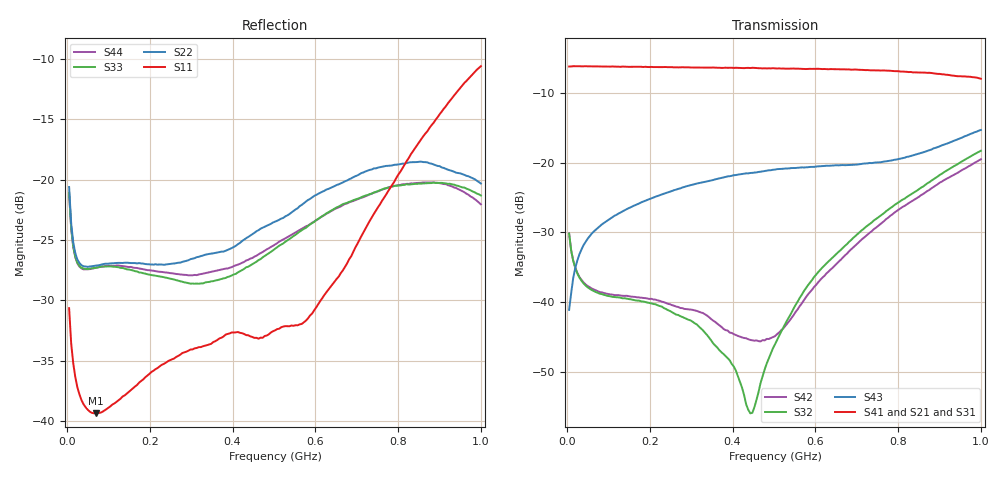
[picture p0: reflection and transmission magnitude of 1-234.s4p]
!Vector Network Analyzer,NA7684A,8000025053,DSP: 1.0.1
!Date: 2021-10-28 16:52
!Data & Calibration Information:
!Freq	S11:SOLT4(ON)	S12:SOLT4(ON)	S13:SOLT4(ON)	S14:SOLT4(ON)
!	S21:SOLT4(ON)	S22:SOLT4(ON)	S23:SOLT4(ON)	S24:SOLT4(ON)
!	S31:SOLT4(ON)	S32:SOLT4(ON)	S33:SOLT4(ON)	S34:SOLT4(ON)
!	S41:SOLT4(ON)	S42:SOLT4(ON)	S43:SOLT4(ON)	S44:SOLT4(ON)
# Hz S dB R 50
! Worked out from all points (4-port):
!   201 points, 5 MHz to 1 GHz, reference 50 ohm
!   strongest paths, dB at 5 MHz, 253.8 MHz, 502.5 MHz, 751.2 MHz, 1 GHz:
!     S41: -6.2, -6.3, -6.5, -6.8, -8.0
!     S21: -6.2, -6.3, -6.6, -6.9, -8.1
!     S31: -6.2, -6.4, -6.6, -7.0, -8.1
!     S43: -41.1, -24.1, -21.0, -20.0, -15.3
!     S32: -30.2, -41.4, -46.0, -27.9, -18.3
!     S42: -30.2, -40.4, -44.9, -29.1, -19.5
!   lowest |S11| = -39.4 dB at 69.67 MHz (marker M1), VSWR 1.02, Z = 50.3 + j1.05 ohm
!   |S11| at or under -10 dB: start of sweep to end of sweep
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5000000  -30.65 121.4  -6.17 0.4  -6.21 0.6  -6.23 0.4
         -6.19 0.2  -20.62 137.4  -30.14 -42.6  -30.16 -42.9
         -6.21 0.0  -30.16 -42.7  -21.08 137.8  -41.11 73.5
         -6.23 -0.2  -30.16 -42.8  -41.10 73.7  -21.14 137.7
6.9675e7  -39.35 75.3  -6.19 -15.5  -6.22 -15.6  -6.20 -15.4
          -6.19 -15.9  -27.12 176.5  -38.40 -20.9  -38.20 -26.0
          -6.21 -16.1  -38.54 -21.2  -27.30 174.8  -29.60 45.4
          -6.22 -16.1  -38.32 -26.0  -29.60 45.2  -27.30 176.2
3.18425e8  -33.88 -34.3  -6.38 -72.6  -6.40 -73.0  -6.36 -72.3
           -6.36 -73.0  -26.39 -164.5  -42.75 -29.5  -41.42 -63.8
           -6.39 -73.5  -43.48 -29.7  -28.62 -169.4  -22.94 27.5
           -6.37 -73.0  -41.36 -65.0  -22.94 27.1  -27.85 -168.5
4.47775e8  -33.03 -87.2  -6.49 -103.4  -6.50 -103.8  -6.46 -103.0
           -6.47 -103.8  -24.51 -155.5  -61.46 35.0  -45.19 -127.2
           -6.48 -104.5  -55.85 51.7  -27.00 -152.9  -21.41 17.5
           -6.42 -103.5  -45.45 -127.4  -21.47 17.2  -26.49 -155.4
4.97525e8  -32.56 -116.7  -6.52 -115.6  -6.55 -115.9  -6.48 -114.8
           -6.50 -116.0  -23.56 -154.0  -47.23 103.5  -44.85 -170.9
           -6.54 -116.7  -46.61 94.5  -25.86 -150.5  -20.97 14.3
           -6.47 -115.6  -45.02 -168.8  -21.02 13.7  -25.49 -152.7
5.9205e8  -31.10 -178.8  -6.66 -139.4  -6.67 -139.7  -6.56 -138.5
          -6.66 -140.1  -21.48 -158.5  -36.77 100.8  -38.11 136.2
          -6.69 -140.6  -36.82 96.8  -23.61 -151.8  -20.53 8.4
          -6.57 -139.6  -38.21 134.4  -20.61 8.1  -23.58 -153.4
1e9  -10.61 -12.8  -8.07 98.3  -8.06 98.3  -7.95 101.9
     -8.10 97.7  -20.32 156.9  -18.27 17.5  -19.48 17.3
     -8.06 97.5  -18.30 18.0  -21.32 164.8  -15.36 0.9
     -7.98 101.4  -19.53 17.6  -15.32 0.3  -22.05 156.6
